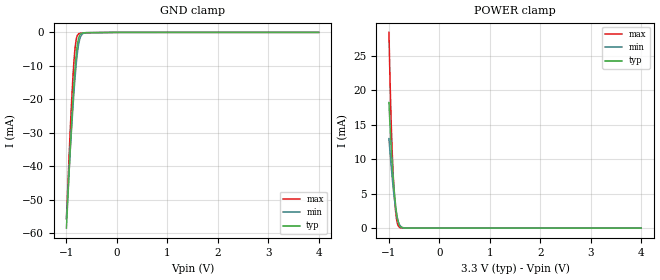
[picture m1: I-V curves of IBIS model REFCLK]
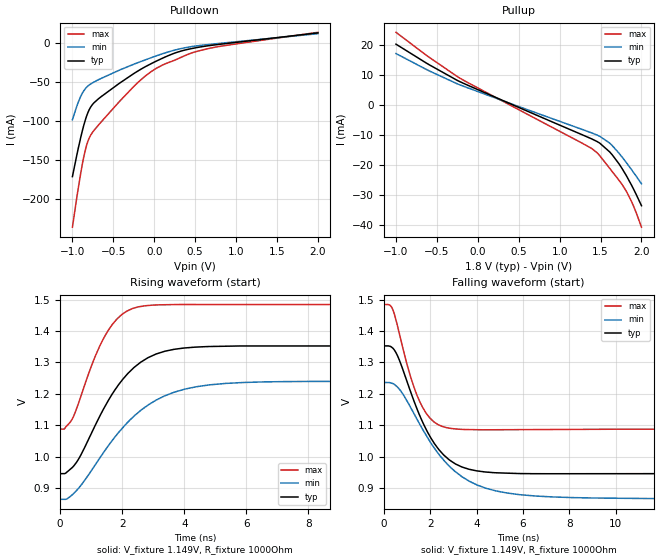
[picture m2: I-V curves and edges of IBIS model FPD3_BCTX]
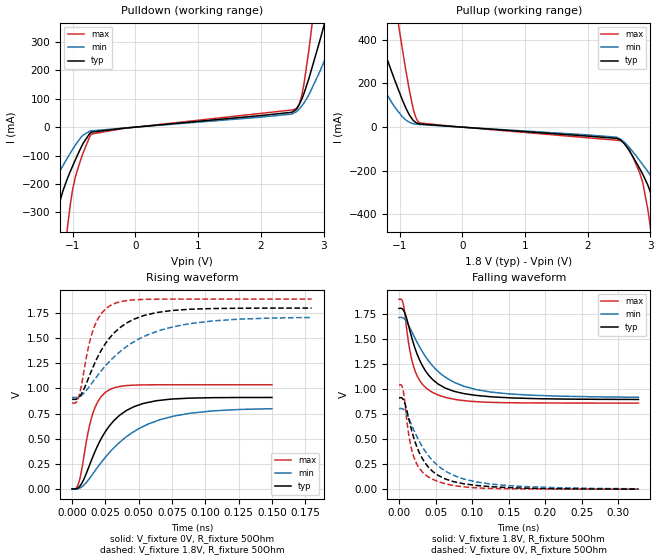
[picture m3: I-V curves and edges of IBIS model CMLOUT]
|Texas Instruments Incorporated
| Marketing part#   Package-type   #pins
| DS90UB662-Q1   VQFN   64
[IBIS Ver]   4.1
[File name]   ds90ub662q1.ibs
[File Rev]   1.0
[Date]   09/16/2020
[Source]
| Texas Instruments Incorporated.
| 12500 TI Blvd
| Dallas, TX -75243
[Notes]   Revision History:
| Rev 1.0: 09/16/2020
| - Initial version
[Disclaimer]
| This model is designed as an aid for customers of Texas Instruments.
| TI and its licensors and suppliers make no warranties, either expressed
| or implied, with respect to this  model, including the warranties of
| merchantability or fitness for a particular purpose. The model is
| provided solely on an "as is" basis. The entire risk as to its quality
| and performance is with the customer.
[Copyright]
 (C) Copyright 2015 Texas Instruments Incorporated.All rights reserved.
|   Device
[Component]   DS90UB662-Q1
[Manufacturer]   TI
[Package]  |QFN   64
|   typ   min   max
R_pkg   0   0   0
L_pkg   0   0   0
C_pkg   0   0   0
[Pin]  signal_name   model_name   R_pin   L_pin   C_pin
1   VDD18_P3   POWER   NA   NA   NA
2   VDD18_P2   POWER   NA   NA   NA
3   PDB   PDB   NA   NA   NA
4   TESTEN   IO_LVCMOS   NA   NA   NA
5   REFCLK   REFCLK   NA   NA   NA
6   INTB   IO_OPEN_DRAIN   NA   NA   NA
7   I2C_SDA2   IO_OPEN_DRAIN   NA   NA   NA
8   I2C_SCL2   IO_OPEN_DRAIN   NA   NA   NA
9   GPIO0   IO_LVCMOS   NA   NA   NA
10   GPIO1   IO_LVCMOS   NA   NA   NA
11   I2C_SDA   IO_OPEN_DRAIN   NA   NA   NA
12   I2C_SCL   IO_OPEN_DRAIN   NA   NA   NA
13   VDDL1   POWER   NA   NA   NA
14   GPIO2   IO_LVCMOS   NA   NA   NA
15   GPIO3   IO_LVCMOS   NA   NA   NA
16   VDDIO   POWER   NA   NA   NA
17   GPIO4   IO_LVCMOS   NA   NA   NA
18   GPIO5   IO_LVCMOS   NA   NA   NA
19   GPIO6   IO_LVCMOS   NA   NA   NA
20   GPIO7   IO_LVCMOS   NA   NA   NA
21   VDD_CSI0   POWER   NA   NA   NA
22   CSI0_CLKN   CSI_DRV   NA   NA   NA
23   CSI0_CLKP   CSI_DRV   NA   NA   NA
24   CSI0_D0N   CSI_DRV   NA   NA   NA
25   CSI0_D0P   CSI_DRV   NA   NA   NA
26   CSI0_D1N   CSI_DRV   NA   NA   NA
27   CSI0_D1P   CSI_DRV   NA   NA   NA
28   CSI0_D2N   CSI_DRV   NA   NA   NA
29   CSI0_D2P   CSI_DRV   NA   NA   NA
30   CSI0_D3N   CSI_DRV   NA   NA   NA
31   CSI0_D3P   CSI_DRV   NA   NA   NA
32   VDD18A   POWER   NA   NA   NA
33   VDD_CSI1   POWER   NA   NA   NA
34   CSI1_CLKN   CSI_DRV   NA   NA   NA
35   CSI1_CLKP   CSI_DRV   NA   NA   NA
36   CSI1_D0N   CSI_DRV   NA   NA   NA
37   CSI1_D0P   CSI_DRV   NA   NA   NA
38   CSI1_D1N   CSI_DRV   NA   NA   NA
39   CSI1_D1P   CSI_DRV   NA   NA   NA
40   CSI1_D2N   CSI_DRV   NA   NA   NA
41   CSI1_D2P   CSI_DRV   NA   NA   NA
42   CSI1_D3N   CSI_DRV   NA   NA   NA
43   CSI1_D3P   CSI_DRV   NA   NA   NA
44   VDDL2   POWER   NA   NA   NA
45   MODE   IO_STRAP   NA   NA   NA
46   IDX   IO_STRAP   NA   NA   NA
47   VDD18_P1   POWER   NA   NA   NA
48   VDD18_P0   POWER   NA   NA   NA
49   VDD18_FPD0   POWER   NA   NA   NA
50   RIN0+   FPD3   NA   NA   NA
51   RIN0-   FPD3   NA   NA   NA
52   VDD_FPD1   POWER   NA   NA   NA
53   RIN1+   FPD3   NA   NA   NA
54   RIN1-   FPD3   NA   NA   NA
55   VDD18_FPD1   POWER   NA   NA   NA
56   CMLOUTP   CMLOUT   NA   NA   NA
57   CMLOUTN   CMLOUT   NA   NA   NA
58   VDD18_FPD2   POWER   NA   NA   NA
59   RIN2+   FPD3   NA   NA   NA
60   RIN2-   FPD3   NA   NA   NA
61   VDD_FPD2   POWER   NA   NA   NA
62   RIN3+   FPD3   NA   NA   NA
63   RIN3-   FPD3   NA   NA   NA
64   VDD18_FPD3   POWER   NA   NA   NA
[Diff Pin]  inv_pin  vdiff  tdelay_typ tdelay_min tdelay_max
23   22   NA   NA   NA   NA
25   24   NA   NA   NA   NA
27   26   NA   NA   NA   NA
29   28   NA   NA   NA   NA
31   30   NA   NA   NA   NA
35   34   NA   NA   NA   NA
37   36   NA   NA   NA   NA
39   38   NA   NA   NA   NA
41   40   NA   NA   NA   NA
43   42   NA   NA   NA   NA
50   51   NA   NA   NA   NA
53   54   NA   NA   NA   NA
59   60   NA   NA   NA   NA
62   63   NA   NA   NA   NA
|   Model Selectors
[Model Selector]  CSI_DRV
CSI_DRV_HS   csi driver in normal mode
CSI_DRV_LP   csi driver in low power mode
[Model Selector]  FPD3
FPD3_RX   FPD3 buffer in receiver model
FPD3_BCTX   FPD3 buffer in driver model
[Model Selector]  IO_LVCMOS
IO_LVCMOS_1p8  input buffer at 1.8V operation.
IO_LVCMOS_3p3  input buffer at 3.3V operation.
[Define Package Model]  dp90ub60pkg
[Manufacturer]  Unknown
[OEM]  Unknown
[Description]  None
[Number Of Pins]  64
[Pin Numbers]
|Pin Num   Terminal Name
1
2
3
4
5
6
7
8
9
10
11
12
13
14
15
16
17
18
19
20
21
22
23
24
25
26
27
28
29
30
31
32
33
34
35
36
37
38
39
40
41
42
43
44
45
46
47
48
49
50
51
52
53
54
55
56
57
58
59
60
61
62
63
64
[Model Data]
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[End Model Data]
[End Package Model]
| Models and submodels in the file (11): REFCLK (Input), FPD3_BCTX (Output), CMLOUT (Output), CSI_DRV_HS (Output), CSI_DRV_LP (Output), FPD3_RX (Input), IO_LVCMOS_1p8 (I/O), IO_LVCMOS_3p3 (I/O), IO_STRAP (Input), IO_OPEN_DRAIN (I/O_open_drain), PDB (Input)
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|   REFCLK Model
[Model]   REFCLK
Model_type   Input
Vinl = 0.99
Vinh = 2.31
|   typ   min   max
C_comp   0.217pF   0.155pF   0.285pF
[Voltage Range]   3.3   3   3.6
[Temperature Range]   27   105   -40
[Power Clamp Reference]   3.3   3   3.6
[GND Clamp Reference]   0   0   0
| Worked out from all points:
|   GND clamp passes 1 mA (typ) near -0.74 V on its own axis
|   POWER clamp passes 1 mA (typ) near -0.82 V on its own axis
[GND Clamp]
|   Voltage   I(typ)   I(min)   I(max)
-1V       -58.46mA   -55.76mA   -55.55mA
-930mV    -36.46mA   -36.76mA   -30.93mA
-910mV    -30.68mA   -31.67mA   -24.51mA
-875mV    -21.25mA   -23.26mA   -14.4mA
-850mV    -15.22mA   -17.76mA   -8.48mA
-825mV    -9.978mA   -12.8mA    -4.141mA
-810mV    -7.323mA   -10.17mA   -2.45mA
-785mV    -3.906mA   -6.458mA   -964.5uA
-755mV    -1.549mA   -3.298mA   -398.4uA
-720mV    -501.1uA   -1.299mA   -238.6uA
-615mV    -84.48uA   -95.6uA    -122.5uA
4V        0A         0A         0A
[POWER Clamp]
|   Voltage   I(typ)   I(min)   I(max)
-1V       18.23mA    12.99mA    28.42mA
-980mV    15.09mA    11.12mA    21.96mA
-955mV    11.73mA    8.928mA    15.27mA
-935mV    9.381mA    7.299mA    11.02mA
-910mV    6.809mA    5.441mA    6.923mA
-880mV    4.227mA    3.534mA    3.455mA
-850mV    2.264mA    2.057mA    1.358mA
-830mV    1.348mA    1.339mA    626.9uA
-800mV    532.9uA    639uA      172.3uA
-740mV    64.05uA    118uA      16.27uA
-665mV    7.756uA    15.09uA    5.838uA
4V        0A         0A         0A
|   FPD3_BCTX Model
[Model]   FPD3_BCTX
Model_type   Output
Polarity   Non-Inverting
Vmeas = 1.6
Vref = 1.8
Cref = 1pF
Rref = 50
|   typ   min   max
C_comp   0.938pF   0.681pF   1.119pF
[Voltage Range]   1.8   1.71   1.89
[Temperature Range]   27   105   -40
[Pullup Reference]   1.8   1.71   1.89
[Pulldown Reference]   -0   0   0
[Power Clamp Reference]   1.8   1.71   1.89
[GND Clamp Reference]   0   0   0
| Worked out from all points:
|   slope of the pulldown table from 0 to 0.27 V, typ, clamps not added: 22 ohm
|   slope of the pullup table from 0 to 0.27 V, typ, clamps not added: 84.2 ohm
|   falling waveform, V_fixture 1.149V, R_fixture 1000Ohm: 20-80 % time 1.47ns typ, 2.2ns min, 976ps max; typ from 1.35 V to 0.946 V
|   rising waveform, V_fixture 1.149V, R_fixture 1000Ohm: 20-80 % time 1.47ns typ, 1.91ns min, 987ps max; typ from 0.946 V to 1.35 V
[Pulldown]
|   Voltage   I(typ)   I(min)   I(max)
-1V       -171.7mA   -98.53mA   -236.6mA
-931mV    -136.5mA   -76.76mA   -188.1mA
-877mV    -112.1mA   -64.18mA   -154.7mA
-838mV    -97.47mA   -58.19mA   -135.7mA
-793mV    -85.34mA   -53.79mA   -121.7mA
-649mV    -68.97mA   -45.52mA   -101.5mA
-250mV    -39.27mA   -27.24mA   -55.84mA
-103mV    -30.11mA   -21.43mA   -41.96mA
35mV      -22.8mA    -16.15mA   -31.93mA
248mV     -13.07mA   -9.187mA   -22.14mA
545mV     -5.396mA   -3.33mA    -10.09mA
2V        13.01mA    11.98mA    13.73mA
[Pullup]
|   Voltage   I(typ)   I(min)   I(max)
-1V       20.31mA    17.19mA    24.25mA
-592mV    13.43mA    11.4mA     15.89mA
-223mV    7.882mA    6.809mA    9.073mA
1.262V    -9.676mA   -7.929mA   -12.44mA
1.391V    -11.2mA    -9.211mA   -14.39mA
1.457V    -12.09mA   -9.937mA   -15.81mA
1.49V     -12.62mA   -10.35mA   -16.8mA
1.637V    -16.34mA   -13.28mA   -21.9mA
1.724V    -19.47mA   -15.93mA   -24.93mA
1.814V    -23.4mA    -19.06mA   -28.59mA
1.904V    -27.96mA   -22.41mA   -33.65mA
2V        -33.45mA   -26.17mA   -40.58mA
[Ramp]
R_load = 1000
|   typ   min   max
dV/dt_r   0.243953/1.46588e-09   0.22325/1.90603e-09   0.237963/9.8707e-10
dV/dt_f   0.243821/1.47149e-09   0.22325/2.20309e-09   0.237891/9.7583e-10
[Falling Waveform]
V_fixture = 1.149V
V_fixture_min = 1.054V
V_fixture_max = 1.285V
R_fixture = 1000Ohm
C_fixture = 0F
|   Time   V(typ)   V(min)   V(max)
0s        1.352V     1.236V     1.484V
389.4ps   1.345V     1.232V     1.468V
670.5ps   1.308V     1.215V     1.392V
1.144ns   1.209V     1.158V     1.257V
1.674ns   1.11V      1.087V     1.157V
2.151ns   1.045V     1.03V      1.111V
2.718ns   996.3mV    977.8mV    1.092V
4.025ns   954.3mV    909.4mV    1.085V
5.88ns    945.9mV    878.5mV    1.086V
20ns      946mV      863.8mV    1.087V
[Rising Waveform]
V_fixture = 1.149V
V_fixture_min = 1.054V
V_fixture_max = 1.285V
R_fixture = 1000Ohm
C_fixture = 0F
|   Time   V(typ)   V(min)   V(max)
0s        945.6mV    863.8mV    1.087V
137.5ps   945.6mV    863.8mV    1.088V
422.9ps   968.4mV    881.4mV    1.126V
1.083ns   1.09V      966.8mV    1.308V
1.553ns   1.179V     1.034V     1.402V
1.978ns   1.241V     1.087V     1.452V
2.519ns   1.295V     1.141V     1.477V
3.677ns   1.342V     1.205V     1.484V
5.331ns   1.351V     1.233V     1.484V
20ns      1.352V     1.236V     1.484V
|   CMLOUT Model
[Model]   CMLOUT
Model_type   Output
Polarity   Non-Inverting
Vmeas = 0.9
Vref = 0
Cref = 2pF
Rref = 70
|   typ   min   max
|   (nom PVT)   (fast PVT)   (slow PVT)
C_comp   6.389e-13   2.780e-13   1.035e-12
| Where nom  PVT is Nominal Process, 1.8V, 27C
|   Fast PVT is Strong Process,  1.89V, -40C
|   Slow PVT is Weak Process,   1.71V, 125C
[Voltage Range]   1.8   1.71   1.89
|Junction Temperature
[Temperature Range]   27   125   -40
[Pullup Reference]   1.8   1.71   1.89
[Pulldown Reference]   0   0   0
[Power Clamp Reference]   1.8   1.71   1.89
[GND Clamp Reference]   0   0   0
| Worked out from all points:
|   slope of the pulldown table from 0 to 0.27 V, typ, clamps not added: 49.1 ohm
|   slope of the pullup table from 0 to 0.27 V, typ, clamps not added: 48.8 ohm
|   falling waveform, V_fixture 1.8V, R_fixture 50Ohm: 20-80 % time 35.4ps typ, 54.4ps min, 21.1ps max; typ from 1.8 V to 0.895 V
|   rising waveform, V_fixture 0V, R_fixture 50Ohm: 20-80 % time 23.8ps typ, 40ps min, 10.4ps max; typ from 0 V to 0.91 V
|   rising waveform, V_fixture 1.8V, R_fixture 50Ohm: 20-80 % time 25.9ps typ, 43.7ps min, 11.6ps max; typ from 0.892 V to 1.8 V
|   falling waveform, V_fixture 0V, R_fixture 50Ohm: 20-80 % time 32.8ps typ, 50.5ps min, 19.4ps max; typ from 0.911 V to 0.003 V
[Pulldown]
|   Voltage   I(typ)   I(min)   I(max)
-1.8V     -847.6mA   -471.7mA   -1.971A
-1.41V    -451.8mA   -239.9mA   -1.064A
-1.269V   -317.2mA   -179.9mA   -744.9mA
-1.086V   -181.3mA   -108.8mA   -356.7mA
-949.5mV  -111mA     -60.46mA   -169mA
-729.5mV  -22.27mA   -14.33mA   -34.04mA
2.502V    52.87mA    46.56mA    60.65mA
2.613V    79.84mA    64.25mA    80.83mA
2.766V    171.3mA    114.1mA    272.1mA
2.933V    298mA      191.7mA    567.5mA
3.207V    521mA      335.9mA    1.087A
3.6V      849mA      551.6mA    1.849A
[Pullup]
|   Voltage   I(typ)   I(min)   I(max)
-1.8V     811.3mA    471.2mA    1.976A
-1.369V   450.7mA    236.1mA    1.136A
-1.077V   215mA      91.56mA    578.4mA
-954mV    123.7mA    47.05mA    354.3mA
-844.2mV  55.93mA    22.27mA    169.1mA
-677.3mV  14.59mA    12.11mA    19.19mA
2.46V     -51.33mA   -46.33mA   -59.89mA
2.723V    -136.6mA   -113.9mA   -138.3mA
2.975V    -278.2mA   -210.3mA   -409.6mA
3.08V     -367.5mA   -253.6mA   -625.6mA
3.29V     -571.5mA   -365.5mA   -1.095A
3.6V      -886.4mA   -561.6mA   -1.811A
[Ramp]
R_load = 50
|   typ   min   max
dV/dt_r   0.546351/2.38441e-11   0.48204/4.06607e-11   0.62238/1.04745e-11
dV/dt_f   0.544765/3.57859e-11   0.47988/5.56984e-11   0.620843/2.13489e-11
[Falling Waveform]
V_fixture = 1.8V
V_fixture_min = 1.71V
V_fixture_max = 1.89V
R_fixture = 50Ohm
|   Time   V(typ)   V(min)   V(max)
0s        1.8V       1.71V      1.89V
3.173ps   1.802V     1.712V     1.891V
5.952ps   1.785V     1.705V     1.84V
14.24ps   1.597V     1.617V     1.407V
22.12ps   1.399V     1.5V       1.176V
35.8ps    1.184V     1.326V     1.019V
53.49ps   1.049V     1.175V     939.6mV
88.77ps   953.4mV    1.027V     884mV
125.8ps   922mV      968.8mV    866.8mV
327.4ps   895.4mV    917.2mV    858.8mV
[Rising Waveform]
V_fixture = 0V
V_fixture_min = 0V
V_fixture_max = 0V
R_fixture = 50Ohm
|   Time   V(typ)   V(min)   V(max)
0s        61.91uV    112.7uV    102.3uV
5.027ps   15.77mV    4.797mV    61.38mV
13.04ps   235.6mV    104.1mV    629.1mV
17.37ps   377.5mV    183.5mV    815.9mV
22.12ps   507mV      268mV      923.8mV
28.55ps   635.7mV    369.5mV    990.8mV
46.4ps    817.8mV    570mV      1.032V
65.93ps   881.1mV    688.2mV    1.036V
105.5ps   907.6mV    776mV      1.036V
150.1ps   909.7mV    797.9mV    1.036V
[Rising Waveform]
V_fixture = 1.8V
V_fixture_min = 1.71V
V_fixture_max = 1.89V
R_fixture = 50Ohm
|   Time   V(typ)   V(min)   V(max)
0s        891.9mV    910mV      855.1mV
5.027ps   909.3mV    915.7mV    917.1mV
11.93ps   1.09V      1V         1.392V
17.37ps   1.262V     1.098V     1.637V
25.06ps   1.446V     1.224V     1.79V
32.92ps   1.569V     1.33V      1.85V
53.61ps   1.724V     1.513V     1.885V
76.15ps   1.776V     1.614V     1.888V
105.5ps   1.794V     1.671V     1.889V
179.9ps   1.799V     1.706V     1.889V
[Falling Waveform]
V_fixture = 0V
V_fixture_min = 0V
V_fixture_max = 0V
R_fixture = 50Ohm
|   Time   V(typ)   V(min)   V(max)
0s        910.9mV    803.8mV    1.038V
3.173ps   912.5mV    805.7mV    1.039V
5.952ps   891.8mV    797.2mV    975.4mV
13.04ps   714.6mV    713mV      557.6mV
19.62ps   527.7mV    601.9mV    337.2mV
31.55ps   312mV      430.5mV    177.9mV
45.12ps   186.4mV    293.7mV    104.3mV
76.15ps   75.48mV    136mV      38.29mV
125.8ps   28.03mV    53.73mV    10.83mV
327.4ps   3.294mV    6.782mV    3.611mV
